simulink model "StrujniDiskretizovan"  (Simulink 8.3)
settings: Solver=ode45  StartTime=0.0  StopTime=Tfinal  MaxStep=50e-6  RelTol=1e-3
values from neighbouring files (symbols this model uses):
  DELTA = 50    [StrujniDiskretizovan_parametri.m]
  Ib = 726    [StrujniDiskretizovan_parametri.m]
  Ki = Kp * K/Tpwm    [StrujniDiskretizovan_parametri.m]
  Ki_a = Kp_a/Tn    [StrujniDiskretizovan_parametri.m]
  Kinv = Vdc/sqrt(3)    [StrujniDiskretizovan_parametri.m]
  Kp = (1-exp(-lambda*T))/(Kps*(exp(T/Tsigma)-1)*(1+n*(1-exp(-lambda*T))))    [StrujniDiskretizovan_parametri.m]
  Kp_a = lambda*Tsigma/(Kinv*Ks/Ib)    [StrujniDiskretizovan_parametri.m]
  Ks = 1/Rs    (= 222.222222222)    [StrujniDiskretizovan_parametri.m]
  T = Tpwm    (= 6.60022440763e-05)    [StrujniDiskretizovan_parametri.m]
  T0 = 0    [StrujniDiskretizovan_parametri.m]
  T1 = 100e-3    (= 0.1)    [StrujniDiskretizovan_parametri.m]
  T2 = 200e-3    (= 0.2)    [StrujniDiskretizovan_parametri.m]
  T3 = 300e-3    (= 0.3)    [StrujniDiskretizovan_parametri.m]
  T4 = 400e-3    (= 0.4)    [StrujniDiskretizovan_parametri.m]
  Tsigma = sigma*Ts    (= 0.0122644628099)    [StrujniDiskretizovan_parametri.m]
  Vh = 70.7    [StrujniDiskretizovan_parametri.m]
  Vl = -70.7    [StrujniDiskretizovan_parametri.m]
undefined symbols (not defined in the file or in its folder): DiscIntNeverNeededParam
libraries: simulink x3

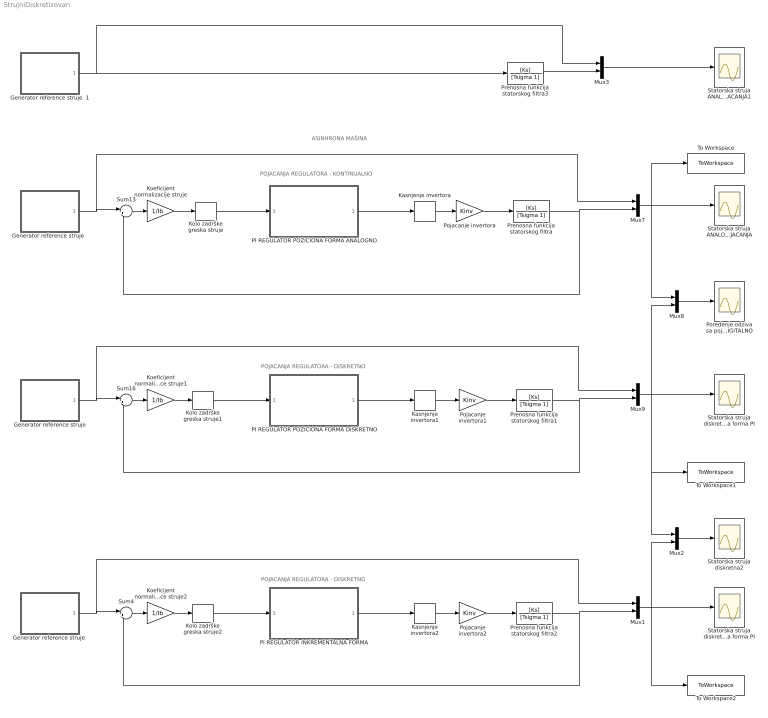
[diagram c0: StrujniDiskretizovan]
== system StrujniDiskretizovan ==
  note: POJACANJA REGULATORA - DISKRETNO
  note: POJACANJA REGULATORA - KONTINUALNO
  note: ASINHRONA MAŠINA
  note: POJACANJA REGULATORA - DISKRETNO
  Generator reference struje : Subsystem
  "Generator reference struje " : Subsystem
  "Generator reference struje  " : Subsystem
  Generator reference struje  1 : Subsystem
  Kasnjenje invertora : Delay  DelayLength=1
  Kasnjenje invertora1 : Delay  DelayLength=1
  Kasnjenje invertora2 : Delay  DelayLength=1  SampleTime=T
  Koeficijent normalizacije reference struje1 : Gain  Gain=1/Ib
  Koeficijent normalizacije reference struje2 : Gain  Gain=1/Ib
  Koeficijent normalizacije struje : Gain  Gain=1/Ib
  Kolo zadrške greska struje : ZeroOrderHold  SampleTime=T
  Kolo zadrške greska struje1 : ZeroOrderHold  SampleTime=T
  Kolo zadrške greska struje2 : ZeroOrderHold  SampleTime=T
  Mux{1..3,7..9} (6 alike) : Mux  Inputs=2
  PI REGULATOR INKREMENTALNA FORMA : Subsystem
  PI REGULATOR POZICIONA FORMA ANALOGNO : Subsystem
  PI REGULATOR POZICIONA FORMA DISKRETNO : Subsystem
  Pojacanje invertora : Gain  Gain=Kinv
  Pojacanje invertora1 : Gain  Gain=Kinv
  Pojacanje invertora2 : Gain  Gain=Kinv
  Poredenje odziva sa pojacanjima regulatora ANALOGNO/DIGITALNO : Scope
  Prenosna funkcija statorskog filtra{,1..3} (4 alike) : TransferFcn  Numerator=[Ks]  Denominator=[Tsigma 1]
  Statorska struja ANALOGNA POJACANJA : Scope
  Statorska struja ANALOGNA POJACANJA1 : Scope
  Statorska struja diskretna Inkrementalna forma PI : Scope
  Statorska struja diskretna Poziciona forma PI : Scope
  Statorska struja diskretna2 : Scope
  Sum13 : Sum  Inputs=|+-
  Sum16 : Sum  Inputs=|+-
  Sum4 : Sum  Inputs=|+-
  To Workspace : ToWorkspace  VariableName=struja_stator  SampleTime=-1
  To Workspace1 : ToWorkspace  VariableName=struja_stator_diskr  SampleTime=-1
  To Workspace2 : ToWorkspace  VariableName=struja_stator_diskr1  SampleTime=-1
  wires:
  Mux7/1 -> Mux8/1, To Workspace/1, Statorska struja ANALOGNA POJACANJA/1
  Kasnjenje invertora/1 -> Pojacanje invertora/1
  Sum13/1 -> Koeficijent normalizacije struje/1
  Mux8/1 -> Poredenje odziva sa pojacanjima regulatora ANALOGNO/DIGITALNO/1
  Mux9/1 -> Mux8/2, Statorska struja diskretna Poziciona forma PI/1, Mux2/1, To Workspace1/1
  Kasnjenje invertora1/1 -> Pojacanje invertora1/1
  Sum16/1 -> Koeficijent normalizacije reference struje1/1
  Prenosna funkcija statorskog filtra1/1 -> Sum16/2, Mux9/2
  Generator reference struje/1(Iref) -> Mux9/1, Sum16/1
  Pojacanje invertora/1 -> Prenosna funkcija statorskog filtra/1
  Prenosna funkcija statorskog filtra/1 -> Sum13/2, Mux7/2
  Pojacanje invertora1/1 -> Prenosna funkcija statorskog filtra1/1
  Koeficijent normalizacije struje/1 -> Kolo zadrške greska struje/1
  Koeficijent normalizacije reference struje1/1 -> Kolo zadrške greska struje1/1
  Mux1/1 -> Mux2/2, To Workspace2/1, Statorska struja diskretna Inkrementalna forma PI/1
  Kasnjenje invertora2/1 -> Pojacanje invertora2/1
  Sum4/1 -> Koeficijent normalizacije reference struje2/1
  Prenosna funkcija statorskog filtra2/1 -> Mux1/2, Sum4/2
  "Generator reference struje "/1(Iref) -> Sum4/1, Mux1/1
  Pojacanje invertora2/1 -> Prenosna funkcija statorskog filtra2/1
  Koeficijent normalizacije reference struje2/1 -> Kolo zadrške greska struje2/1
  PI REGULATOR INKREMENTALNA FORMA/1(Vref) -> Kasnjenje invertora2/1
  Kolo zadrške greska struje2/1 -> PI REGULATOR INKREMENTALNA FORMA/1(e)
  Kolo zadrške greska struje1/1 -> PI REGULATOR POZICIONA FORMA DISKRETNO/1(e)
  Kolo zadrške greska struje/1 -> PI REGULATOR POZICIONA FORMA ANALOGNO/1(e)
  Mux2/1 -> Statorska struja diskretna2/1
  "Generator reference struje  "/1(Iref) -> Sum13/1, Mux7/1
  PI REGULATOR POZICIONA FORMA ANALOGNO/1(Vref) -> Kasnjenje invertora/1
  PI REGULATOR POZICIONA FORMA DISKRETNO/1(Vref) -> Kasnjenje invertora1/1
  Mux3/1 -> Statorska struja ANALOGNA POJACANJA1/1
  Generator reference struje  1/1(Iref) -> Prenosna funkcija statorskog filtra3/1, Mux3/1
  Prenosna funkcija statorskog filtra3/1 -> Mux3/2

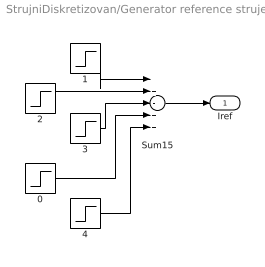
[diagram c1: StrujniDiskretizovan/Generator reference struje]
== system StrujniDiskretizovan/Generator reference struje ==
  0 : Step  Time=T0  After=DELTA  SampleTime=0
  1 : Step  Time=T1  After=DELTA  SampleTime=0
  2 : Step  Time=T2  After=DELTA  SampleTime=0
  3 : Step  Time=T3  After=DELTA  SampleTime=0
  4 : Step  Time=T4  After=DELTA  SampleTime=0
  Sum15 : Sum  Inputs=|+-++-
  Iref : Outport
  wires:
  Sum15/1 -> Iref/1
  3/1 -> Sum15/3
  2/1 -> Sum15/2
  4/1 -> Sum15/5
  0/1 -> Sum15/4
  1/1 -> Sum15/1

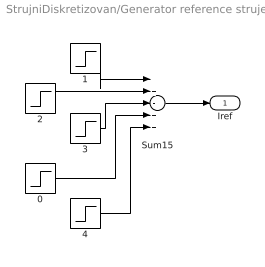
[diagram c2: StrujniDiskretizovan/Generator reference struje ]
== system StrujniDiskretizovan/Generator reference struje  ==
  0 : Step  Time=T0  After=DELTA  SampleTime=0
  1 : Step  Time=T1  After=DELTA  SampleTime=0
  2 : Step  Time=T2  After=DELTA  SampleTime=0
  3 : Step  Time=T3  After=DELTA  SampleTime=0
  4 : Step  Time=T4  After=DELTA  SampleTime=0
  Sum15 : Sum  Inputs=|+-++-
  Iref : Outport
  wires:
  1/1 -> Sum15/1
  0/1 -> Sum15/4
  4/1 -> Sum15/5
  2/1 -> Sum15/2
  3/1 -> Sum15/3
  Sum15/1 -> Iref/1

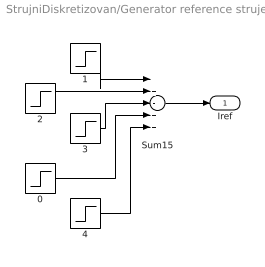
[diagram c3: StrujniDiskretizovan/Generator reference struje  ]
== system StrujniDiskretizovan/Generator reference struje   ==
  0 : Step  Time=T0  After=DELTA  SampleTime=0
  1 : Step  Time=T1  After=DELTA  SampleTime=0
  2 : Step  Time=T2  After=DELTA  SampleTime=0
  3 : Step  Time=T3  After=DELTA  SampleTime=0
  4 : Step  Time=T4  After=DELTA  SampleTime=0
  Sum15 : Sum  Inputs=|+-++-
  Iref : Outport
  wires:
  1/1 -> Sum15/1
  0/1 -> Sum15/4
  4/1 -> Sum15/5
  2/1 -> Sum15/2
  3/1 -> Sum15/3
  Sum15/1 -> Iref/1

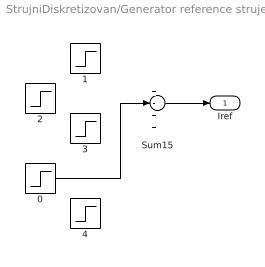
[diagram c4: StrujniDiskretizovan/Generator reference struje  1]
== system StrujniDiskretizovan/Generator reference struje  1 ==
  0 : Step  Time=T0  SampleTime=0
  1 : Step  Time=T1  After=DELTA  SampleTime=0
  2 : Step  Time=T2  After=DELTA  SampleTime=0
  3 : Step  Time=T3  After=DELTA  SampleTime=0
  4 : Step  Time=T4  After=DELTA  SampleTime=0
  Sum15 : Sum  Inputs=|+-++-
  Iref : Outport
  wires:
  Sum15/1 -> Iref/1
  0/1 -> Sum15/3

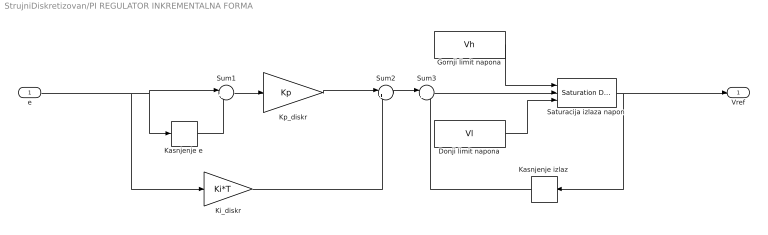
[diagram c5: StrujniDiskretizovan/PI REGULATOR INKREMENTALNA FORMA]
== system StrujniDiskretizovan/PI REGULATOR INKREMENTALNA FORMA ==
  e : Inport
  Donji limit napona : Constant  Value=Vl  SampleTime=T
  Gornji limit napona : Constant  Value=Vh  SampleTime=T
  Kasnjenje izlaz : Delay  DelayLength=1  SampleTime=T
  Kasnjenje e : Delay  DelayLength=1  SampleTime=T
  Ki_diskr : Gain  Gain=Ki*T  SampleTime=T
  Kp_diskr : Gain  Gain=Kp  SampleTime=T
  Saturacija izlaza napon : simulink/Discontinuities/Saturation Dynamic  OutMin=[]  OutMax=[]  OutDataTypeStr=Inherit: Same as second input  OutDataType=fixdt(1, 16)  OutScaling=2^-10  DoSatur=off
  Sum1 : Sum  Inputs=|+-  SampleTime=T
  Sum2 : Sum  Inputs=|++  SampleTime=T
  Sum3 : Sum  Inputs=|++  SampleTime=T
  Vref : Outport
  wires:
  Gornji limit napona/1 -> Saturacija izlaza napon/1
  e/1 -> Sum1/1, Kasnjenje e/1, Ki_diskr/1
  Donji limit napona/1 -> Saturacija izlaza napon/3
  Sum1/1 -> Kp_diskr/1
  Ki_diskr/1 -> Sum2/2
  Kp_diskr/1 -> Sum2/1
  Sum2/1 -> Sum3/1
  Sum3/1 -> Saturacija izlaza napon/2
  Kasnjenje izlaz/1 -> Sum3/2
  Saturacija izlaza napon/1 -> Vref/1, Kasnjenje izlaz/1
  Kasnjenje e/1 -> Sum1/2

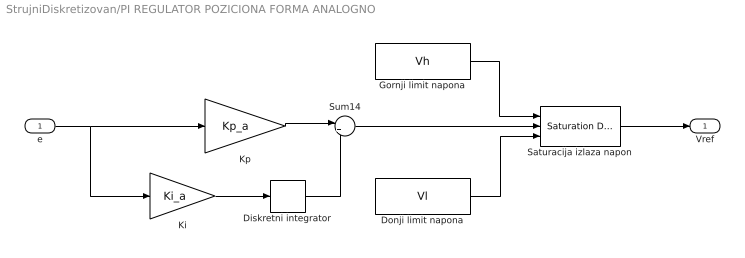
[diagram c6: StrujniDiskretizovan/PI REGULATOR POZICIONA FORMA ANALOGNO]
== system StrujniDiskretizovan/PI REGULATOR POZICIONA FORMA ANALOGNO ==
  e : Inport
  Diskretni integrator : DiscreteIntegrator  IntegratorMethod=Integration: Backward Euler  SampleTime=T  ICPrevOutput=DiscIntNeverNeededParam  ICPrevScaledInput=DiscIntNeverNeededParam
  Donji limit napona : Constant  Value=Vl  SampleTime=T
  Gornji limit napona : Constant  Value=Vh  SampleTime=T
  Ki : Gain  Gain=Ki_a
  Kp : Gain  Gain=Kp_a
  Saturacija izlaza napon : simulink/Discontinuities/Saturation Dynamic  OutMin=[]  OutMax=[]  OutDataTypeStr=Inherit: Same as second input  OutDataType=fixdt(1, 16)  OutScaling=2^-10  DoSatur=off
  Sum14 : Sum  Inputs=|++
  Vref : Outport
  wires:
  Kp/1 -> Sum14/1
  Ki/1 -> Diskretni integrator/1
  Diskretni integrator/1 -> Sum14/2
  e/1 -> Kp/1, Ki/1
  Gornji limit napona/1 -> Saturacija izlaza napon/1
  Donji limit napona/1 -> Saturacija izlaza napon/3
  Sum14/1 -> Saturacija izlaza napon/2
  Saturacija izlaza napon/1 -> Vref/1

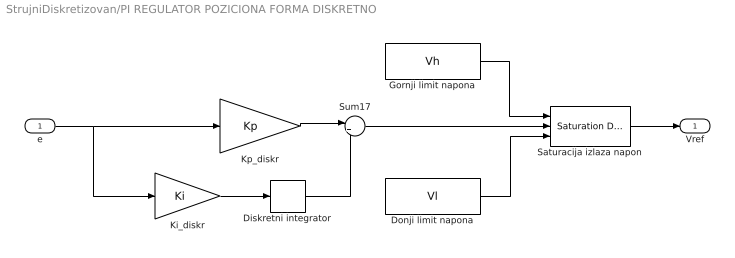
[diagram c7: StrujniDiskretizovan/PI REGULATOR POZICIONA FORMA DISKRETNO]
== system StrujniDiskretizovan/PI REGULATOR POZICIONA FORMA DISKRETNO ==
  e : Inport
  Diskretni integrator : DiscreteIntegrator  IntegratorMethod=Integration: Backward Euler  SampleTime=T  ICPrevOutput=DiscIntNeverNeededParam  ICPrevScaledInput=DiscIntNeverNeededParam
  Donji limit napona : Constant  Value=Vl  SampleTime=T
  Gornji limit napona : Constant  Value=Vh  SampleTime=T
  Ki_diskr : Gain  Gain=Ki
  Kp_diskr : Gain  Gain=Kp
  Saturacija izlaza napon : simulink/Discontinuities/Saturation Dynamic  OutMin=[]  OutMax=[]  OutDataTypeStr=Inherit: Same as second input  OutDataType=fixdt(1, 16)  OutScaling=2^-10  DoSatur=off
  Sum17 : Sum  Inputs=|++
  Vref : Outport
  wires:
  Kp_diskr/1 -> Sum17/1
  Ki_diskr/1 -> Diskretni integrator/1
  Diskretni integrator/1 -> Sum17/2
  e/1 -> Kp_diskr/1, Ki_diskr/1
  Gornji limit napona/1 -> Saturacija izlaza napon/1
  Donji limit napona/1 -> Saturacija izlaza napon/3
  Sum17/1 -> Saturacija izlaza napon/2
  Saturacija izlaza napon/1 -> Vref/1
